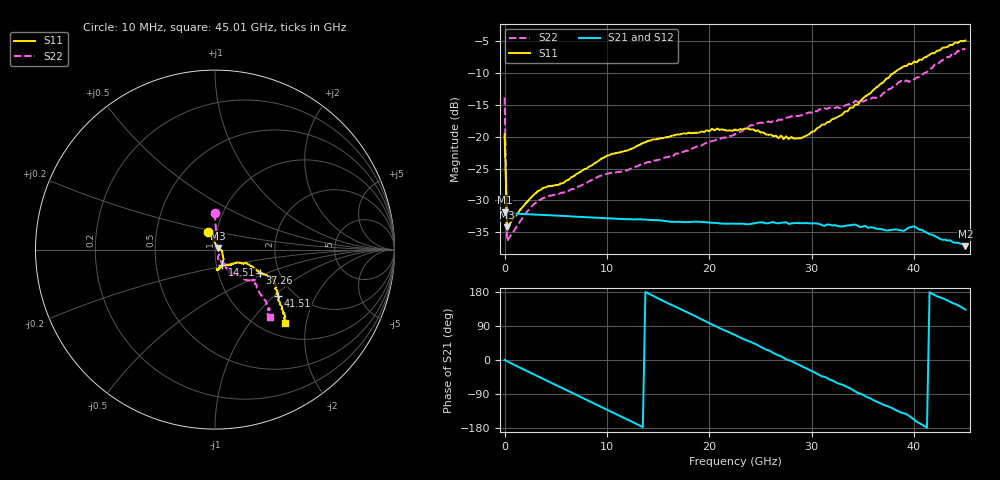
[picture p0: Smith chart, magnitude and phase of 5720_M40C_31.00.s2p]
! Device:  ADRF5720
! Description: 0.5dB LSB GaAs MMIC 6-bit Digital Attenuator
! Frequency:  0.000009 -  40 GHz
! Ports:
!	RF1	= Port 1
!	RF2	= Port 2
! Vdd:  3.3 Volt
! Vss:  -3.3 Volt
! Control:  0/3.3 Volt
! State:  31.00 dB attenuation
! Data:  The device was measured using G-S-G Probes on a matrix board.
!  Data was collected using an calibrated 4 port network analyzer.
!  The reference plane for this measurement is at the launchers.
! Note:  Analog Devices supplies this data as a sample of measured data
!  for this product.  Your particular data for this product may vary.
!  Data was taken at -40 degrees C.
!  Analog Devices reserves the right to change this data at anytime.
# GHZ S DB R 45.0
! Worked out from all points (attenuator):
!   181 points, 10 MHz to 45.01 GHz, reference 45 ohm
!   highest |S21| = -31.85 dB at 10 MHz (marker M1); lowest = -37.1 dB at 45.01 GHz (marker M2)
!   lowest |S11| = -34.2 dB at 260 MHz (marker M3), VSWR 1.04, Z = 46.5 + j0.899 ohm
!   |S11| at or under -10 dB: start of sweep to 38.07 GHz
!   |S22| runs from -36.4 to -6.3 dB; largest |S21 - S12| = 0.00015
!   S11 on the Smith chart (normalised r, x): 10 MHz: 0.91, +0.18; 14.51 GHz: 1.06, -0.19; 37.26 GHz: 1.59, -0.45; 41.51 GHz: 1.66, -1.06; 45.01 GHz: 1.26, -1.51
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0.01  -19.63 110.8  -31.85 0.5  -31.86 0.5  -13.89 90.4
0.26  -34.22 29.8  -32.02 -3.6  -32.04 -3.6  -36.37 33.1
3.26  -28.54 -7.6  -32.23 -43.1  -32.25 -43.2  -30.04 -32.0
5.76  -27.27 -23.3  -32.42 -75.6  -32.44 -75.6  -28.78 -52.0
7.76  -25.14 -37.8  -32.59 -101.5  -32.61 -101.6  -27.41 -65.9
10.01  -22.99 -47.9  -32.79 -130.9  -32.81 -131.0  -25.83 -69.9
14.51  -20.44 -65.9  -33.06 169.3  -33.08 169.2  -23.72 -68.7
15.26  -20.27 -68.4  -33.12 159.0  -33.14 158.9  -23.55 -67.4
20.26  -18.82 -81.7  -33.48 93.8  -33.50 93.7  -20.73 -58.8
22.76  -19.06 -85.3  -33.64 62.8  -33.66 62.7  -19.51 -59.2
24.01  -18.92 -80.8  -33.68 48.1  -33.70 48.0  -18.25 -58.0
27.76  -20.40 -68.3  -33.68 -0.7  -33.71 -0.9  -16.96 -55.9
30.26  -19.17 -48.8  -33.57 -32.5  -33.60 -32.7  -15.97 -57.2
32.76  -16.75 -29.2  -34.07 -63.4  -34.11 -63.5  -15.57 -53.2
34.76  -14.39 -22.7  -34.17 -89.1  -34.19 -89.1  -14.25 -49.2
37.26  -10.99 -27.6  -34.69 -120.6  -34.71 -120.8  -13.05 -46.1
37.76  -10.28 -27.2  -34.61 -125.8  -34.63 -126.1  -12.50 -44.8
38.76  -9.25 -25.9  -34.69 -139.1  -34.70 -139.4  -11.30 -40.3
40.01  -8.26 -29.3  -34.06 -157.6  -34.04 -157.8  -11.06 -38.7
41.51  -7.20 -36.2  -35.29 178.9  -35.30 178.6  -9.44 -43.5
43.76  -5.65 -42.4  -36.51 150.1  -36.52 149.8  -6.88 -47.7
45.01  -4.97 -46.3  -37.15 133.2  -37.19 132.9  -6.30 -50.9
